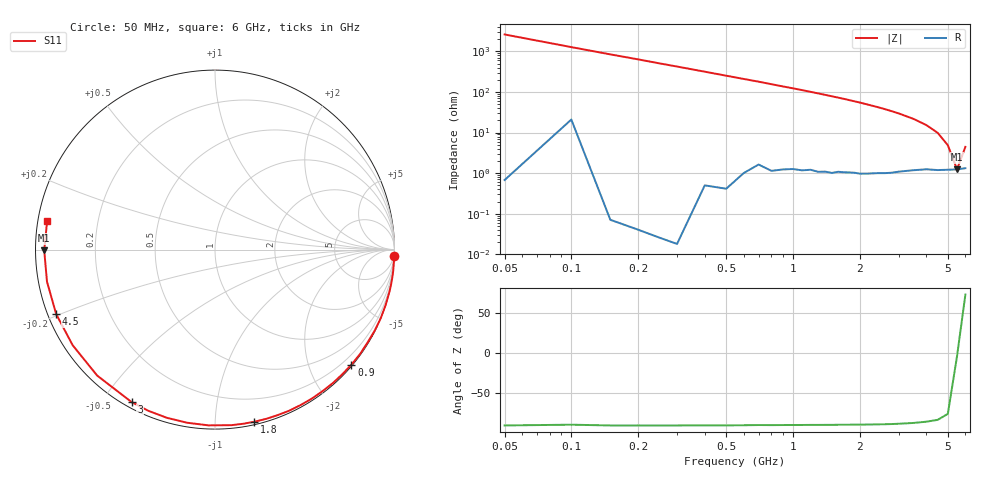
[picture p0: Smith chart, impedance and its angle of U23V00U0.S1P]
! SIEMENS Discrete & RF Semiconductors
! BBY52-02W
! Si Tuning Diode in SCD-80
! VR = 3 V
! S-Parameters:  September  1997
# GHz  S  MA  R  50
!  f  S11
! GHz  MAG  ANG
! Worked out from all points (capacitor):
!   34 points, 50 MHz to 6 GHz, reference 50 ohm
!   read as one part to ground: C = 1.25 pF near 50 MHz
!   lowest |Z| = 1.24 ohm at 5.5 GHz (marker M1)
!   series resonance near 5.51 GHz, so ESL is about 670 pH
!   S11 on the Smith chart (normalised r, x): 50 MHz: 0, -52; 900 MHz: 0.02, -2.74; 1.8 GHz: 0.02, -1.25; 3 GHz: 0.02, -0.59; 4.5 GHz: 0.02, -0.20; 6 GHz: 0.03, +0.08
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0.05  1 -2.2
0.2  1 -9.0
0.3  1 -13.5
0.4  0.9995 -18.0
0.5  0.9994 -22.5
0.6  0.9978 -26.9
0.7  0.9953 -31.2
0.8  0.9957 -35.7
0.9  0.9942 -40.1
1.1  0.9921 -48.5
1.2  0.9905 -52.8
1.3  0.9902 -57.0
1.5  0.9883 -65.2
1.6  0.9861 -69.2
1.7  0.9852 -73.0
1.8  0.9839 -77.1
2  0.9825 -84.6
2.2  0.9799 -92.1
2.4  0.9771 -99.1
2.6  0.9748 -105.9
2.8  0.972 -112.5
3  0.9682 -118.7
3.5  0.961 -133.1
4  0.9554 -146.1
4.5  0.9551 -157.9
5  0.953 -169.2
5.5  0.9516 -179.8
6  0.9487 170.3
